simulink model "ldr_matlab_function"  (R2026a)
settings: Solver=FixedStepAuto  StopTime=inf  EnableMultiTasking=on
libraries: arduinolib x2

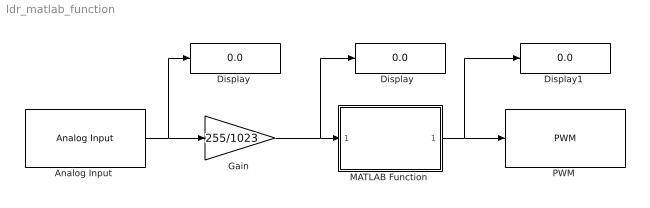
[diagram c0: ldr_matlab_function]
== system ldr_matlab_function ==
  "Analog Input " : arduinolib/Analog Input  pinNumber=0  ReadResultsOnly=off  ConversionTriggerSource=Software  ExternalTriggerType=uint32( 0 )  OutputDataType=uint16  EnableConversionCompleteNotify=off  EnableOuputStatus=off  SampleTime=0.01  blockPlatform=arduino
  "Display " : Display
  "Display  " : Display
  "Display1 " : Display
  "Gain " : Gain  Gain=255/1023
  "MATLAB Function " : MATLAB Function  TreatAsAtomicUnit=on
  "PWM " : arduinolib/PWM  pinNumber=9  frequencyType=Default  desiredFrequency=490.2  achievableFrequency=490.2
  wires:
  "Analog Input "/1 -> "Gain "/1, "Display "/1
  "Gain "/1 -> "Display  "/1, "MATLAB Function "/1(u)
  "MATLAB Function "/1(y) -> "Display1 "/1, "PWM "/1

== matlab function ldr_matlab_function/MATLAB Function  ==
function y = fcn(u) 
if u <= cast(255/2,'like',u) 
y = u; 
else 
y = cast(0,'like',u); 
end
